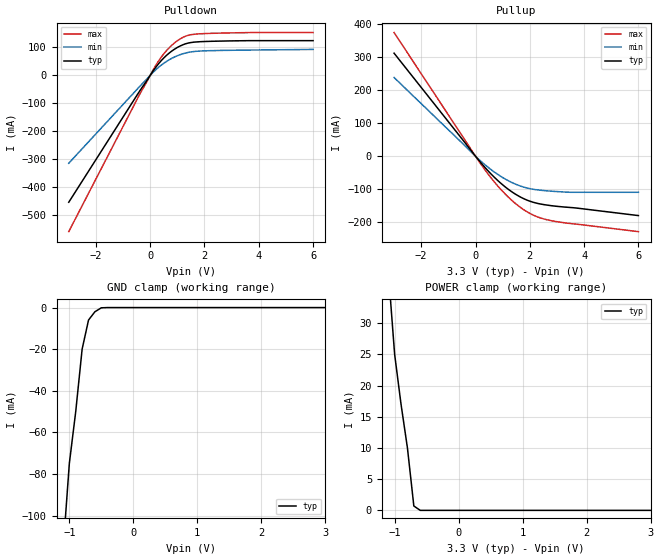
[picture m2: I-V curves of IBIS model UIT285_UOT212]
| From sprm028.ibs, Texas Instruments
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[Model]   UIT285_UOT212
Model_type   I/O
Polarity   Non-Inverting
Enable   Active-Low
| signals   A, GZ, Y
Vinl = 0.8V
Vinh = 2.0V
Cref = 30p
Rref = 50
Vref = 1.5
Vmeas = 1.5
|   typ   min   max
C_comp   3.6757p   3.5409p   3.8618p
|   typ   min   max
[Temperature Range]   25.0   0   90
|   typ   min   max
[Voltage Range]   3.3V   3.13V   3.47V
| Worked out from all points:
|   slope of the pulldown table from 0 to 0.495 V, typ, clamps not added: 8.03 ohm
|   slope of the pullup table from 0 to 0.495 V, typ, clamps not added: 10.5 ohm
|   GND clamp passes 1 mA (typ) near -0.55 V on its own axis
|   POWER clamp passes 1 mA (typ) near -0.70 V on its own axis
[Pulldown]
|   Voltage   I(typ)   I(min)   I(max)
-3V       -453.7mA   -314.3mA   -558.8mA
-400mV    -57.75mA   -41.01mA   -70mA
100mV     14.76mA    10.15mA    18.29mA
300mV     40.66mA    28.14mA    50.33mA
500mV     62.19mA    43.3mA     76.94mA
900mV     93.94mA    66.03mA    116.4mA
1.3V      112.9mA    79.93mA    140.1mA
1.7V      119.5mA    86.08mA    147.8mA
3.7V      124.2mA    90.56mA    153.1mA
6V        124.2mA    92.86mA    153.2mA
[GND_clamp]
|   Voltage   I(typ)   I(min)   I(max)
-3V       -900mA     NA         NA
-2V       -500mA     NA         NA
-1V       -75mA      NA         NA
-900mV    -50mA      NA         NA
-800mV    -20mA      NA         NA
-700mV    -6mA       NA         NA
-600mV    -2mA       NA         NA
-500mV    -120uA     NA         NA
-400mV    0A         NA         NA
3V        0A         NA         NA
[Pullup]
|   Voltage   I(typ)   I(min)   I(max)
-3V       312mA      238.3mA    374.4mA
300mV     -29.5mA    -22.31mA   -35.71mA
900mV     -79.43mA   -59.29mA   -97.43mA
1.2V      -99.55mA   -73.74mA   -123.1mA
1.5V      -116.2mA   -85.35mA   -145.1mA
1.8V      -129.3mA   -93.99mA   -163.2mA
2.1V      -138.7mA   -99.61mA   -177.1mA
2.7V      -148.6mA   -105.2mA   -193.5mA
3.5V      -155.2mA   -109.1mA   -203.7mA
6V        -179.6mA   -109.1mA   -228.2mA
[POWER_clamp]
|   Voltage   I(typ)   I(min)   I(max)
-3V       300mA      NA         NA
-2V       160mA      NA         NA
-1V       25mA       NA         NA
-900mV    17mA       NA         NA
-800mV    10mA       NA         NA
-700mV    700uA      NA         NA
-600mV    0A         NA         NA
-500mV    0A         NA         NA
3V        0A         NA         NA
[Ramp]
|   I(typ)   I(min)   I(max)
dV/dt_r   1.711/0.150n   1.513/0.200n   1.853/0.130n
dV/dt_f   1.632/0.140n   1.454/0.210n   1.774/0.100n
